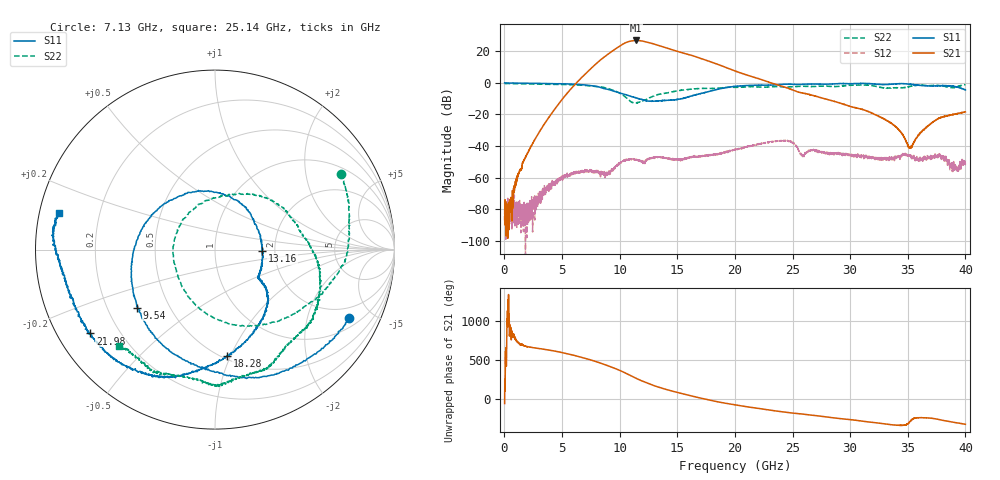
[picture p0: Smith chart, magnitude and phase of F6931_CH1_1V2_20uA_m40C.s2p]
!Keysight Technologies,M9807A,MY58100526,A.15.20.05
!Date: Friday, October 27, 2023 09:15:16
!Correction: S11(C  2-Port  )
!S21(C  2-Port  )
!S12(C  2-Port  )
!S22(C  2-Port  )
!S2P File: Measurements: S11, S21, S12, S22:
# Hz S  dB  R 50
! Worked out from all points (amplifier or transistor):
!   4000 points, 10 MHz to 40 GHz, reference 50 ohm
!   highest |S21| = 26.8 dB at 11.42 GHz (marker M1)
!   |S21| within 3 dB of that: 10.11 GHz to 13.29 GHz (3.179 GHz wide, 27.2 % of centre)
!   unconditionally stable (mu >= 1): start of sweep to 130.3 MHz; 149.7028 MHz to 150.2971 MHz; 179.7 MHz to end of sweep
!   at 6.67 GHz: K = 15.73, MAG = 14.5 dB, |S12| = -55.9 dB
!   at 20.01 GHz: K = 5.05, MAG = 14.8 dB, |S12| = -42.2 dB
!   at 40 GHz: K = 167.70, MAG = -9.9 dB, |S12| = -49.2 dB
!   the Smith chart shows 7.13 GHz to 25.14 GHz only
!   S11 on the Smith chart (normalised r, x): 7.13 GHz: 1.43, -3.67; 9.54 GHz: 0.33, -0.30; 13.16 GHz: 1.71, -0.03; 18.28 GHz: 0.53, -0.97; 21.98 GHz: 0.10, -0.30; 25.14 GHz: 0.06, +0.12
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1e7  -0.02 179.6  -84.77 -56.3  -83.12 77.5  -0.45 180.0
6.68e9  -1.17 -10.4  3.17 172.1  -56.61 72.3  -1.52 40.8
7.13e9  -1.52 -26.8  6.39 153.7  -55.33 60.3  -1.73 30.7
8.39e9  -3.03 -84.6  14.82 95.5  -58.03 -24.0  -2.62 0.3
9.54e9  -5.35 -143.3  20.97 33.4  -53.74 -155.4  -5.04 -40.9
1.001e10  -6.45 -167.8  23.27 4.9  -50.85 165.6  -6.63 -65.2
1.053e10  -7.51 163.0  25.38 -30.5  -48.33 124.8  -9.22 -102.2
1.102e10  -8.71 130.8  26.45 -65.9  -48.07 100.9  -12.19 -150.3
1.142e10  -9.51 102.6  26.77 -94.3  -48.32 77.5  -12.69 162.3
1.186e10  -10.48 68.0  26.50 -124.3  -49.44 69.4  -11.80 117.5
1.223e10  -11.24 41.1  25.95 -147.2  -50.03 72.4  -10.76 88.9
1.316e10  -11.60 -1.8  24.09 163.0  -47.03 44.4  -7.77 44.0
1.334e10  -11.49 -7.9  23.67 154.4  -46.85 40.6  -7.40 37.5
1.429e10  -10.94 -28.9  21.49 112.9  -47.80 16.3  -6.15 10.4
1.568e10  -9.61 -35.3  18.45 60.5  -47.39 4.7  -4.46 -13.2
1.828e10  -4.52 -83.4  12.22 -26.9  -45.01 -28.6  -3.54 -51.5
2.001e10  -2.24 -113.5  7.48 -72.4  -42.16 -46.8  -2.85 -73.1
2.198e10  -1.55 -146.1  2.79 -117.0  -38.81 -95.7  -2.59 -94.7
2.514e10  -0.97 166.6  -4.84 -179.2  -38.16 133.7  -2.40 -134.9
2.667e10  -0.80 146.8  -7.83 156.2  -41.88 128.6  -2.35 -148.8
3.334e10  -0.92 36.3  -24.45 39.2  -48.29 0.5  -3.22 126.7
4e10  -4.43 -131.0  -18.38 39.9  -49.15 -41.2  -1.08 8.4
